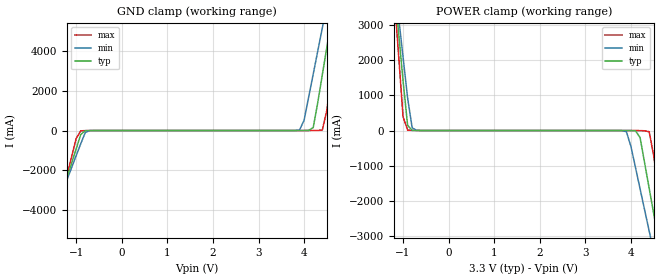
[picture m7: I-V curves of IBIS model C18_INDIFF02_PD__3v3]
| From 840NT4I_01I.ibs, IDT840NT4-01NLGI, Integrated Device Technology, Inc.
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[Model] C18_INDIFF02_PD__3v3
Model_type   Input
Polarity   Non-Inverting
Vinl = 0.8V
Vinh = 2.0V
|   typ   min   max
C_comp   2pF   1.5pF   2.5pF
|   typ   min   max
[Voltage range]   3.3V   3.135V   3.465V
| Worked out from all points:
|   GND clamp passes 1 mA (typ) near -0.68 V on its own axis
|   POWER clamp passes 1 mA (typ) near -0.64 V on its own axis
[GND_clamp]
|Voltage   I (typ)   I (min)   I (max)
-3.3V     -17.55A    -15.11A    -21.66A
-1.7V     -5.988A    -5.48A     -6.879A
-1.5V     -4.541A    -4.276A    -5.028A
-900mV    -200.8mA   -666.1mA   -14.92mA
-700mV    -1.238mA   -4.684mA   -1.66mA
3.9V      486.2uA    26.32mA    87.81uA
4.2V      147.2mA    2.842A     2.963mA
4.4V      2.811A     5.169A     26.53mA
4.6V      5.607A     7.497A     2.804A
4.7V      7.005A     8.661A     4.592A
4.8V      8.403A     9.826A     6.38A
6.6V      33.64A     30.86A     38.61A
[Power_clamp]
|Voltage   I (typ)   I (min)   I (max)
-3.3V     33.64A     28.92A     41.58A
-1.2V     4.209A     4.413A     3.966A
-1.1V     2.811A     3.249A     2.179A
-1V       1.414A     2.086A     391.9mA
-900mV    147.2mA    923.6mA    11.41mA
-700mV    1.726mA    4.468mA    2.147mA
3.9V      -212.6uA   -33.07mA   -11.28uA
4.2V      -200.8mA   -1.658A    -2.709mA
4.4V      -1.646A    -2.861A    -35.09mA
4.6V      -3.093A    -4.065A    -1.65A
4.8V      -4.541A    -5.269A    -3.501A
6.6V      -17.55A    -16.1A     -20.14A
